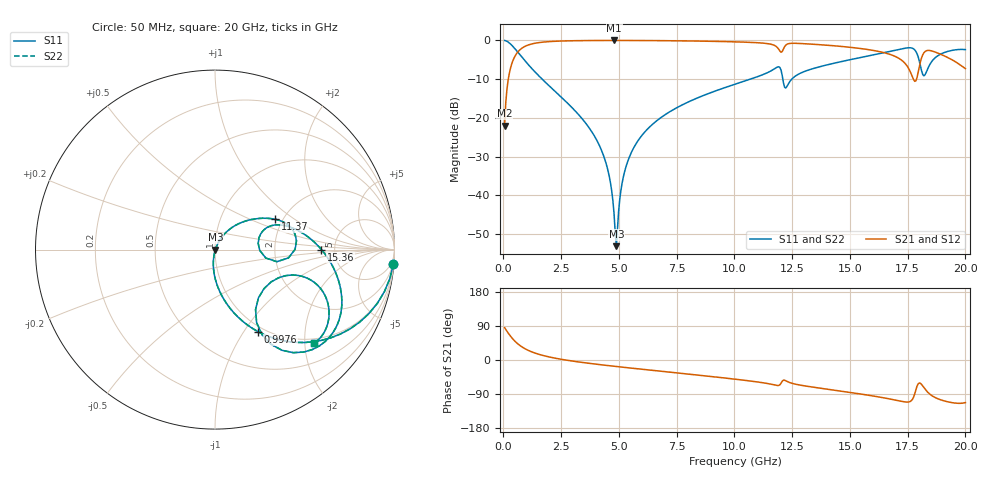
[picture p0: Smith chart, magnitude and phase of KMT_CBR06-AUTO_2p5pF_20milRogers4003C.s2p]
! Data measured by Modelithics Inc. support@modelithics.com 813-866-6335
! KEMET CBR06-AUTO 2.5pF, Pad Width= 0.851mm, Pad Length= 0.64mm, Pad Gap= 0.62mm, 20mil Rogers 4003C substrate Data, January 2022
# hz S ma R 50
! 2 Port Network Data from SP1.SP block
! freq  magS11  angS11  magS21  angS21  magS12  angS12  magS22  angS22
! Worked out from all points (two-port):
!   401 points, 50 MHz to 20 GHz, reference 50 ohm
!   highest |S21| = -0.02 dB at 4.788 GHz (marker M1); lowest = -22.0 dB at 50 MHz (marker M2)
!   |S21| within 3 dB of the highest: 619.6 MHz to 12.01 GHz (11.39 GHz wide, 180 % of centre); 12.03 GHz to 16.37 GHz (4.342 GHz wide, 30.6 % of centre)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
!   lowest |S11| = -53.1 dB at 4.888 GHz (marker M3), VSWR 1.00, Z = 50.2 - j0.0367 ohm
!   |S11| at or under -10 dB: 1.676 GHz to 10.69 GHz (9.013 GHz wide, 146 % of centre); 12.1 GHz to 12.48 GHz (388.1 MHz wide, 3.16 % of centre)
!   |S22| runs from -53.1 to 0.0 dB; largest |S21 - S12| = 0
!   S11 on the Smith chart (normalised r, x): 50 MHz: 1, -24; 997.6 MHz: 0.93, -1.17; 11.37 GHz: 1.83, +0.72; 15.36 GHz: 3.91, +0.00; 20 GHz: 0.90, -2.21
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5e7  0.9968 -4.7  0.07933 85.3  0.07933 85.3  0.9968 -4.7
3.4925e8  0.8726 -30.4  0.4873 59.5  0.4873 59.5  0.8726 -30.4
9.97625e8  0.5174 -62.2  0.8544 27.6  0.8544 27.6  0.5174 -62.2
3.391625e9  0.09889 -95.2  0.9931 -6.3  0.9931 -6.3  0.09889 -95.2
4.389125e9  0.02926 -99.6  0.9973 -13.7  0.9973 -13.7  0.02926 -99.6
4.6385e9  0.0143 -96.8  0.9976 -15.5  0.9976 -15.5  0.0143 -96.8
4.788125e9  0.005832 -84.6  0.9976 -16.5  0.9976 -16.5  0.005832 -84.6
4.887875e9  0.002221 -9.5  0.9976 -17.2  0.9976 -17.2  0.002221 -9.5
5.187125e9  0.01711 63.2  0.9974 -19.2  0.9974 -19.2  0.01711 63.2
5.4365e9  0.03051 64.8  0.997 -20.8  0.997 -20.8  0.03051 64.8
6.73325e9  0.09683 59.3  0.9924 -29.1  0.9924 -29.1  0.09683 59.3
1.0025e10  0.2721 38.5  0.9576 -50.6  0.9576 -50.6  0.2721 38.5
1.137162e10  0.3763 26.6  0.9133 -61.4  0.9133 -61.4  0.3763 26.6
1.206988e10  0.3517 -11.0  0.7194 -56.0  0.7194 -56.0  0.3517 -11.0
1.336662e10  0.4292 17.4  0.893 -71.3  0.893 -71.3  0.4292 17.4
1.536162e10  0.593 0.0  0.7923 -88.8  0.7923 -88.8  0.593 0.0
1.670825e10  0.7178 -15.2  0.6636 -102.6  0.6636 -102.6  0.7178 -15.2
1.78055e10  0.7549 -49.2  0.2965 -89.5  0.2965 -89.5  0.7549 -49.2
1.810475e10  0.4035 -55.9  0.5987 -64.7  0.5987 -64.7  0.4035 -55.9
1.835412e10  0.4202 -20.2  0.741 -84.2  0.741 -84.2  0.4202 -20.2
1.885288e10  0.6467 -21.4  0.6768 -103.4  0.6768 -103.4  0.6467 -21.4
2e10  0.7593 -43.3  0.4323 -112.3  0.4323 -112.3  0.7593 -43.3
